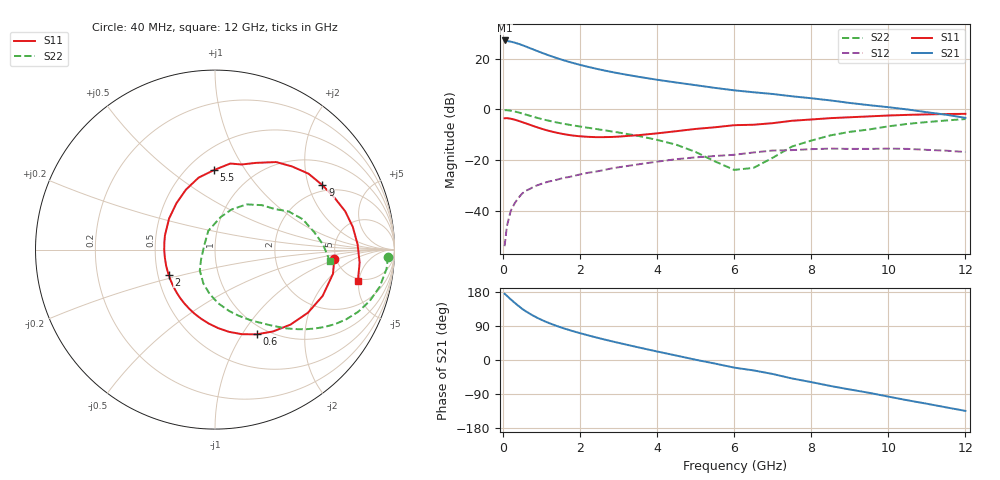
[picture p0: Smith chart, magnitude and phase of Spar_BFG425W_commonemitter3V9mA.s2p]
! Filename: 39bfg425.001
! BFG425W Field C1
! V1=8.379E-001V,V2=3.000E+000V, I1=1.134E-004A, I2=9.010E-003A
# GHz  S  MA  R 50
!  S11  S21  S12  S22
!Freq(GHz)  Mag  Ang  Mag  Ang  Mag  Ang  Mag  Ang
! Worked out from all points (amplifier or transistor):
!   44 points, 40 MHz to 12 GHz, reference 50 ohm
!   highest |S21| = 27.2 dB at 40 MHz (marker M1)
!   |S21| within 3 dB of that: start of sweep to 692.1 MHz
!   unconditionally stable (mu >= 1): 1.976 GHz to end of sweep
!   at 700 MHz: K = 0.50, MSG = 27.8 dB, |S12| = -31.4 dB
!   at 2.4 GHz: K = 1.10, MAG = 18.4 dB, |S12| = -24.6 dB
!   at 12 GHz: K = 1.40, MAG = 3.0 dB, |S12| = -16.8 dB
!   S11 on the Smith chart (normalised r, x): 40 MHz: 4.82, -0.92; 600 MHz: 0.89, -1.16; 2 GHz: 0.57, -0.17; 5.5 GHz: 0.67, +0.73; 9 GHz: 1.77, +2.48; 12 GHz: 4.67, -4.85
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0.04  0.667 -4.6  22.85 174.9  0.002 65.3  0.965 -2.4
0.2  0.653 -23.3  21.64 159.8  0.01 76.1  0.941 -12.7
0.3  0.626 -34.2  20.7 151.2  0.014 71.9  0.908 -18.4
0.4  0.593 -44.8  19.62 142.8  0.018 67.3  0.869 -23.6
0.5  0.559 -54.7  18.46 134.7  0.022 63.2  0.827 -28.1
0.6  0.526 -63.8  17.24 127.9  0.025 60.0  0.785 -32.0
0.8  0.465 -80.3  15.01 116.0  0.03 54.9  0.708 -38.4
0.9  0.438 -87.6  14.02 110.7  0.032 53.1  0.675 -41.1
1.2  0.375 -107.7  11.52 97.2  0.038 49.0  0.594 -47.7
1.4  0.345 -119.6  10.23 89.7  0.041 47.2  0.55 -51.2
1.6  0.322 -131.1  9.164 82.8  0.045 45.6  0.515 -54.5
2  0.294 -151.6  7.535 70.7  0.052 42.8  0.458 -60.9
2.2  0.287 -161.4  6.908 65.2  0.056 41.3  0.434 -64.1
3  0.29 164.1  5.135 45.2  0.072 34.3  0.349 -77.3
3.5  0.309 145.8  4.404 33.6  0.082 28.9  0.3 -86.5
4.5  0.371 116.0  3.38 11.6  0.104 16.0  0.2 -108.9
5.5  0.443 90.8  2.649 -9.4  0.12 1.6  0.094 -145.4
6.5  0.497 72.6  2.174 -27.4  0.141 -9.4  0.07 140.5
8.5  0.671 39.1  1.498 -68.6  0.168 -46.0  0.307 55.1
9  0.698 30.9  1.337 -77.8  0.166 -54.3  0.36 43.5
10.5  0.778 9.4  0.993 -106.3  0.166 -81.3  0.517 19.2
12  0.815 -12.3  0.68 -134.2  0.144 -111.8  0.644 -5.8
